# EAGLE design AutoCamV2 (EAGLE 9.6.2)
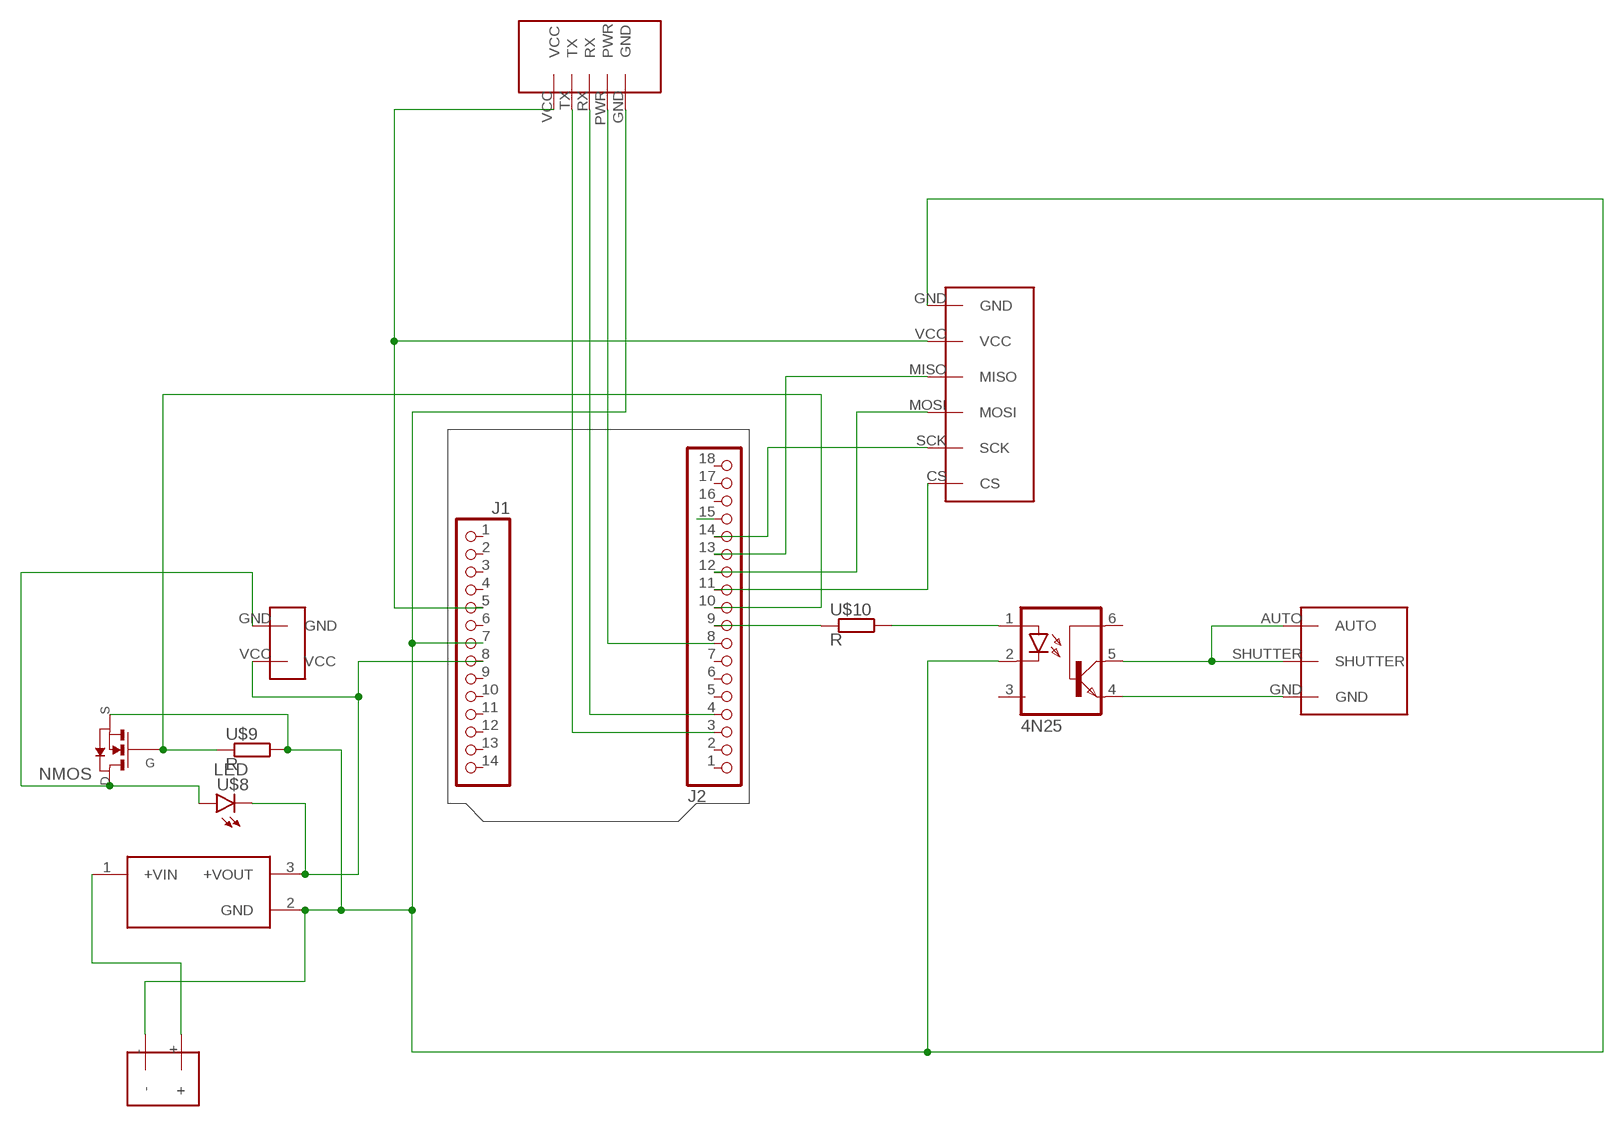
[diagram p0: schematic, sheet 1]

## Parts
J1  -  PINHD-1X14-CUSTOM  [1X14-CUSTOM]
J2  -  PINHD-1X18  [1X18-CUSTOM]
TSRN  TSRN_1-2418A  [CONV_TSRN_1-2418A]
U$1  4N25  [4N25_FOOT]
U$2  SHUTTER_RELEASE  [SHUTTER_RELEASE]
U$3  SS6  [SS6]
U$4  NMOS_RFP12N10L  [N_MOSFET]
U$5  DC_COUPLER  [DC_COUPLER]
U$6  SD  [SD]
U$7  GPS  [GPS]
U$8  LED  [LED]
U$9  R  [R]
U$10  R  [R]

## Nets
N$1 [gnd]: J2.15
N$2: U$1.1(ANODE) U$10.P$1
N$3: U$1.4(EMI) U$2.GND
N$4: J2.13 U$6.MISO
N$5: TSRN.1(+VIN) U$3.+
N$6: J2.9 U$10.P$2
N$7: J1.7 TSRN.2(GND) U$1.2(COTH) U$3.- U$4.S U$6.GND U$7.GND U$9.P$1
N$8: J1.8 TSRN.3(+VOUT) U$5.VCC U$8.P$2(N)
N$9: J2.10 U$4.G U$9.P$2
N$10: U$4.D U$5.GND U$8.P$1(P)
N$11: U$1.5(COL) U$2.AUTO U$2.SHUTTER
N$12: J2.14 U$6.SCK
N$14: J2.12 U$6.MOSI
N$15: J2.11 U$6.CS
N$16: J2.3 U$7.TX
N$17: J2.4 U$7.RX
N$18: J2.8 U$7.PWR
N$19: J1.5 U$6.VCC U$7.VCC
Unconnected: J1.1 J1.2 J1.3 J1.4 J1.6 J1.9 J1.10 J1.11 J1.12 J1.13 J1.14 J2.1 J2.2 J2.5 J2.6 J2.7 J2.16 J2.17 J2.18 U$1.3(NC) U$1.6(BOSE)

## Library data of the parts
J1 = Arduino-connectors:PINHD-1X14: PIN HEADER; DATASHEET: -; DISTRIBUTOR-PN: -; MANUFACTURER: -; MANUFACTURER-PN: -
J2 = Arduino-connectors:PINHD-1X18; DATASHEET: -; DISTRIBUTOR-LINK: -; DISTRIBUTOR-PN: -; MANUFACTURER-PN: -; MANUFCATURER: -
TSRN = TSRN_1-2418A:TSRN_1-2418A: Check availability; AVAILABILITY: In Stock; DESCRIPTION: 1 Amp POL switching regulator, 4.6 to 36 VDC input, pos.-neg. circuit, LM78 compatible, SIP-3; MF: Traco Power; MP: TSRN 1-2418A; PACKAGE: SIP-3 Traco Power; PRICE: None; PURCHASE-URL: https://pricing.snapeda.com/search/part/TSRN 1-2418A/?ref=eda
U$1 = project1:4N25
U$2 = project1:SHUTTER_RELEASE
U$3 = project1:SS6
U$4 = project1:NMOS_RFP12N10L
U$5 = project1:DC_COUPLER
U$6 = project1:SD
U$7 = project1:GPS
U$8 = project1:LED
U$9 U$10 = project1:R

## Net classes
0 default: width 0.254 mm, clearance 0.254 mm
1 power: width 0.61 mm, drill 0.61 mm, clearance 0.254 mm
2 gnd: width 0.305 mm, drill 0.559 mm, clearance 0.254 mm
3 usbvcc: width 0.508 mm, drill 0.61 mm, clearance 0.254 mm
4 aref: width 0.406 mm, drill 0.61 mm, clearance 0.254 mm

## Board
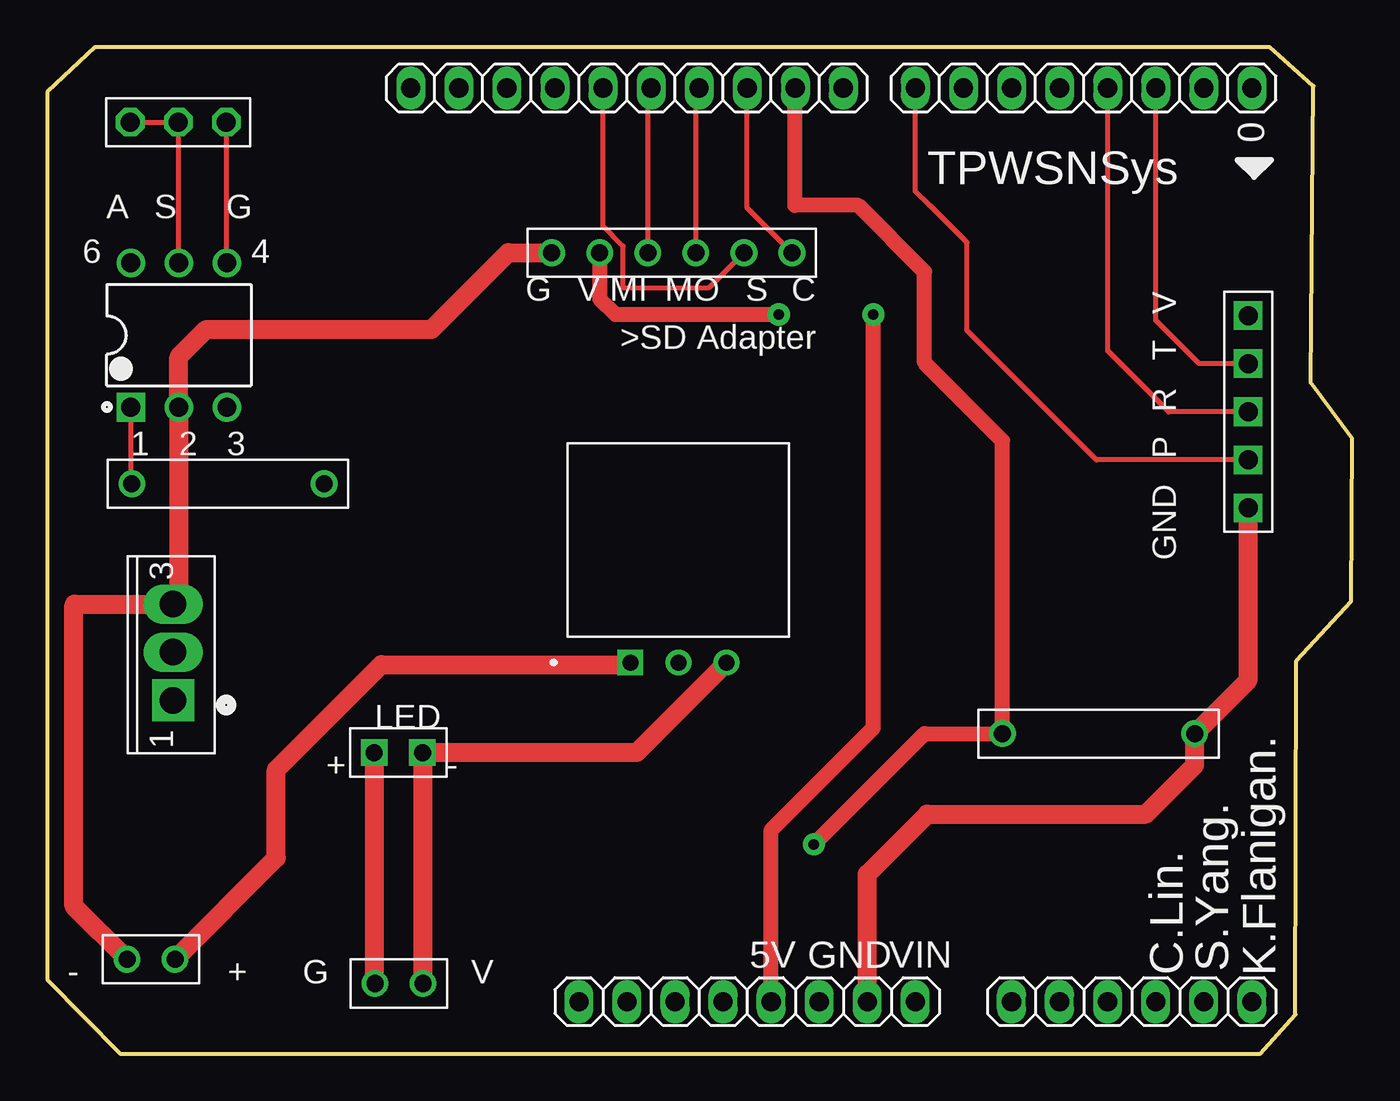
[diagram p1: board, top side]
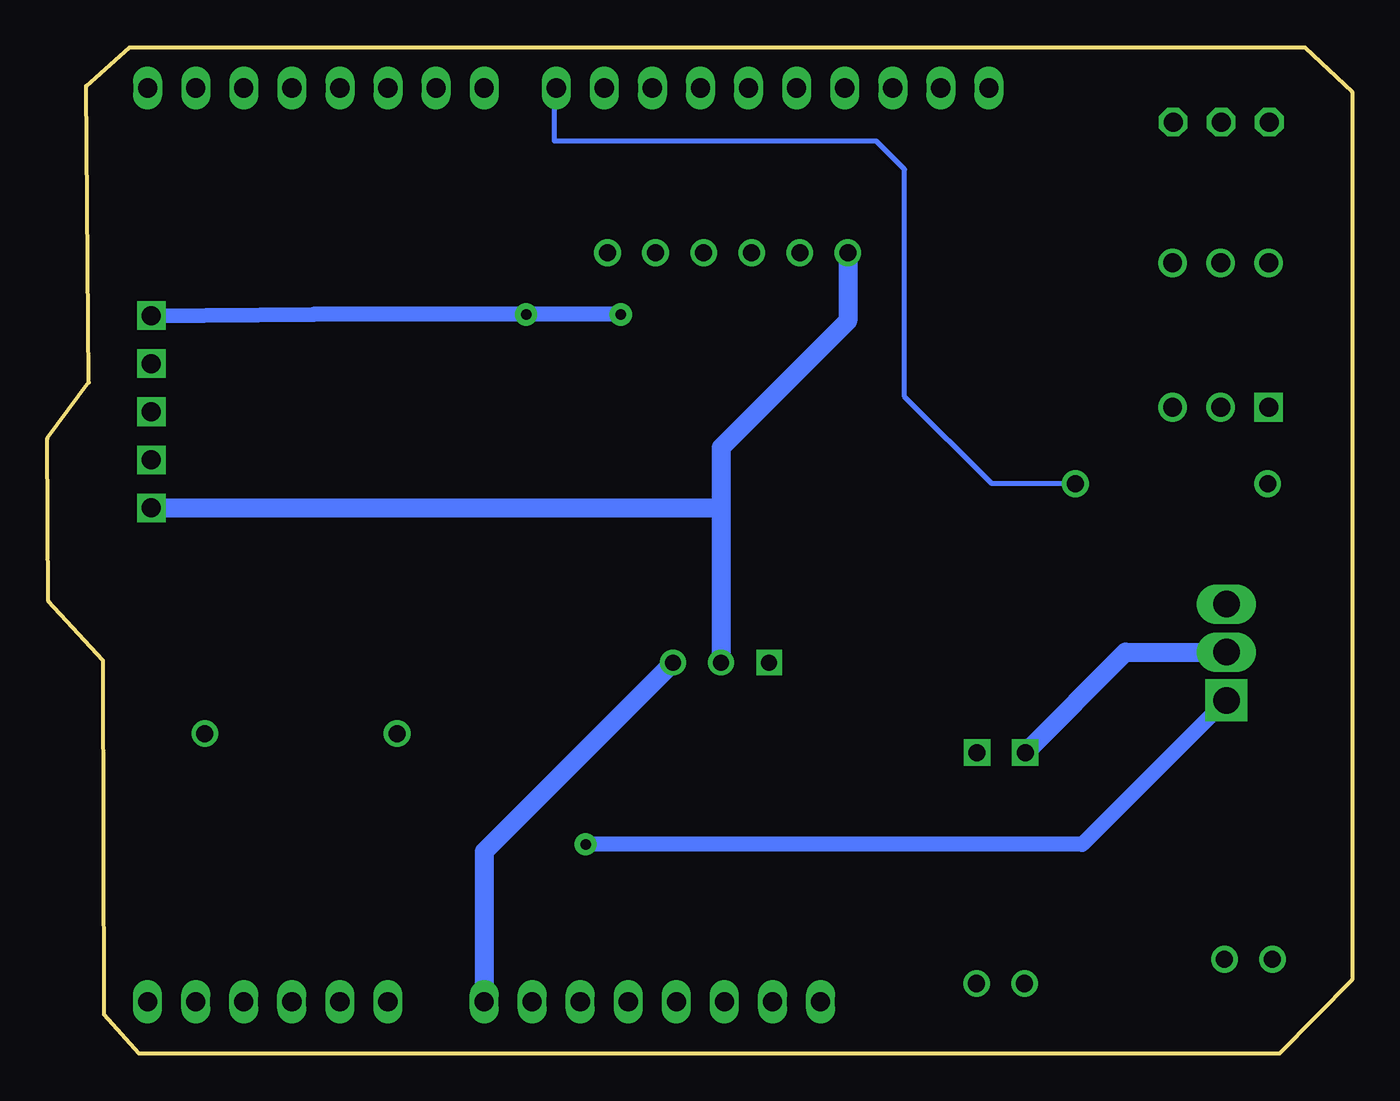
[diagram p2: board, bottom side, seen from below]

Size 68.95 x 53.15 mm. Coordinates in mm from the lower left corner, seen from the top.
Outline: 0,50.8 0,3.9 3.85,0 64.1,0 65.95,2.05 66,20.75 68.9,23.9 68.95,32.5 66.75,35.45 66.9,51.1 64.6,53.15 2.5,53.15 0,50.8
Copper layers (1*16): Top 0.035mm / dielectric 1.5mm / Bottom 0.035mm
Design rules "ArduinoUno *": minimum track width 10mil, minimum drill 22mil, track to track 10mil, track to pad 10mil, pad to pad 10mil, via to via 12mil, smd to smd 8mil, copper to edge 10mil, drill to drill 10mil, minimum pad ring 10mil, minimum via ring 12mil, stop-mask expansion 1mil, vias tented up to drill 30mil, thermal gap 10mil
bKeepout: area 0,3.4 to 2.1,11.2
bRestrict: 5 lines
vRestrict: area 23,44.3 to 24.8,49.3; area 25.5,45.7 to 27.2,49.3; area 28.6,45.5 to 29.7,49; area 31.1,45.5 to 32.3,49; area 33.7,45.5 to 34.8,49; area 36.2,45.5 to 37.4,49; area 38.9,47.4 to 40,49; area 40.4,45.3 to 47.8,47.1; area 60.5,44.4 to 61.9,46.9; area 63,44.4 to 64.4,46.9; area 61.5,36 to 64.9,37.4; area 0.8,22 to 2.2,30.3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

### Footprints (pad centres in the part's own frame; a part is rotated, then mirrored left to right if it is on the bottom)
1X14-CUSTOM = drill 1.016 pad 1.27 long: 1 -17.78,0; 2 -15.24,0; 3 -12.7,0; 4 -10.16,0; 5 -7.62,0; 6 -5.08,0; 7 -2.54,0; 8 0,0; 9 5.08,0; 10 7.62,0; 11 10.16,0; 12 12.7,0; 13 15.24,0; 14 17.78,0
1X18-CUSTOM = drill 1.016 pad 1.27 long: 1 -17.78,0; 2 -15.24,0; 3 -12.7,0; 4 -10.16,0; 5 -7.62,0; 6 -5.08,0; 7 -2.54,0; 8 0,0; 9 3.81,0; 10 6.35,0; 11 8.89,0; 12 11.43,0; 13 13.97,0; 14 16.51,0; 15 19.05,0; 16 21.59,0; 17 24.13,0; 18 26.67,0
CONV_TSRN_1-2418A = drill 0.85 square: 1 2.54,0 | drill 0.85: 2 0,0; 3 -2.54,0
4N25_FOOT = drill 1.001 square: 1 -2.54,-3.81 | drill 1.001: 2 0,-3.81; 3 2.54,-3.81; 4 2.54,3.81; 5 0,3.81; 6 -2.54,3.81
SHUTTER_RELEASE = drill 1 octagon: AUTO -1.27,0; GND 3.81,0; SHUTTER 1.27,0
SS6 = drill 0.9: + 0,1.27; - 2.54,1.27
N_MOSFET = drill 1.4 pad 1.473 long: D 0,0; S 2.54,0 | drill 1.4 pad 2.235 square: G -2.54,0
DC_COUPLER = drill 0.9: GND -2.54,0; VCC 0,0
SD = drill 0.9: CS -6.35,0; GND 6.35,0; MISO 1.27,0; MOSI -1.27,0; SCK -3.81,0; VCC 3.81,0
GPS = drill 1 square: GND 5.08,0; PWR 2.54,0; RX 0,0; TX -2.54,0; VCC -5.08,0
LED = drill 0.9 square: P$1 -1.27,0; P$2 1.27,0
R = drill 0.9: P$1 -5.08,0; P$2 5.08,0

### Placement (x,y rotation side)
J1  45.87,2.74 0 top
J2  45.87,51 180 top
TSRN  33.35,20.65 180 top
U$1  6.95,37.95 0 top
U$2  5.65,49.2 0 top
U$3  6.75,6.25 180 top
U$4  6.65,21.2 90 top
U$5  19.85,3.7 0 top
U$6  33,42.3 180 top
U$7  63.45,33.9 270 top
U$8  18.55,15.9 0 top
U$9  55.55,16.9 180 top
U$10  9.55,30.1 0 top

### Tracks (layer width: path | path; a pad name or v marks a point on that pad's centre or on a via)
N$2
  Top 0.254: U$1.1 4.41,30.16 U$10.P$1
N$3
  Top 0.254: U$2.GND 9.46,41.79 U$1.4
N$4
  Top 0.254: U$6.MISO 31.73,50.83 J2.13
N$5
  Top 1: U$3.+ 12.1,10.33 12.1,15 17.65,20.55 30.71,20.55 TSRN.1
N$6
  Bottom 0.254: U$10.P$2 19.05,30.1 23.65,34.7 23.65,46.7 25.15,48.2 42.15,48.2 42.15,50.91 J2.9
N$7
  Top 1: U$7.GND 63.45,19.72 U$9.P$1 60.63,15.23 58.05,12.65 46.5,12.65 43.33,9.48 J1.7 | U$6.GND 24.35,42.3 20.3,38.25 8.4,38.25 6.95,36.8 U$1.2 6.95,24.04 U$4.S 1.44,23.74 1.4,23.7 1.4,7.79 U$3.-
  Bottom 1: U$6.GND 26.65,38.7 33.35,32 33.35,28.85 | 33.35,28.85 TSRN.2 | U$7.GND 33.38,28.82 33.35,28.85
N$8
  Top 1: U$5.VCC 19.82,3.73 U$8.P$2 31.14,15.9 TSRN.3
  Bottom 1: TSRN.3 45.87,10.67 J1.8
N$9  (via drill 0.56)
  Top 0.8: v40.5,11.05 46.35,16.9 U$9.P$2 50.47,32.38 46.35,36.5 46.35,41.3 42.85,44.8 39.5,44.8 39.5,50.98 J2.10
  Bottom 0.8: U$4.G 14.26,11.05 v40.5,11.05
N$10
  Top 1: U$8.P$1 17.28,3.73 U$5.GND
  Bottom 1: U$8.P$1 11.98,21.2 U$4.D
N$11
  Top 0.254: U$2.AUTO U$2.SHUTTER 6.92,41.79 U$1.5
N$12
  Top 0.254: J2.14 29.36,43.71 30.42,42.65 30.42,40.43 34.93,40.43 U$6.SCK
N$14
  Top 0.254: U$6.MOSI 34.27,50.83 J2.12
N$15
  Top 0.254: U$6.CS 36.98,44.67 J2.11
N$16
  Top 0.254: U$7.TX 60.86,36.44 58.57,38.73 J2.3
N$17
  Top 0.254: U$7.RX 59.25,33.9 56.03,37.12 J2.4
N$18
  Top 0.254: U$7.PWR 55.44,31.36 48.6,38.2 48.6,42.85 46.65,44.8 46.6,44.8 45.87,45.53 J2.8
N$19  (via drill 0.56)
  Top 0.8: U$6.VCC 29.19,39.85 30,39.04 v38.65,39.04 | J1.5 38.25,11.8 43.65,17.2 v43.65,39.04
  Bottom 0.8: v38.65,39.04 v43.65,39.04 54.89,39.04 54.9,39.04 U$7.VCC

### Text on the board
tPlace: 0
tNames: TPWSNSys | 5V | GND | VIN | C.Lin. | S.Yang. | K.Flanigan.
ReferenceLC: L | TX | ON | RX | PC1 | PC2
214bmp: D:/SmartProjects/Snc/a4_bn_logo2.bmp

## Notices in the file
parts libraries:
Arduino-connectors: Copyright (c) 2016-2017 Arduino LLC. All right reserved.
